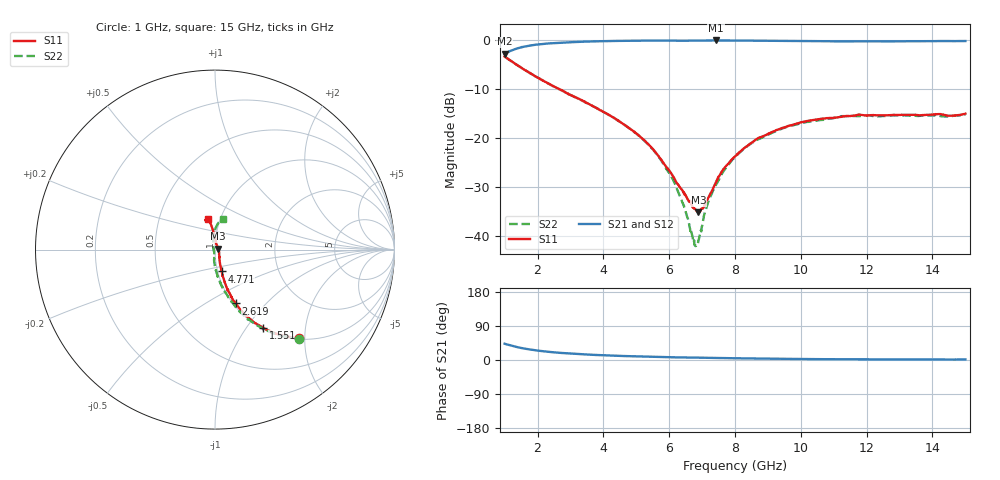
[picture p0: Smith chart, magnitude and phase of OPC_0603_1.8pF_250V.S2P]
! FILE NAME
! DATE 08/20/2012  14:18
! CORRECTED  DATA
# GHz  S  MA  R  50.00
!  FREQ  S11M  S11A  S21M  S21A  S12M  S12A  S22M  S22A
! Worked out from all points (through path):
!   1601 points, 1 GHz to 15 GHz, reference 50 ohm
!   highest |S21| = -0.04 dB at 7.423 GHz (marker M1); lowest = -2.8 dB at 1 GHz (marker M2)
!   group delay of S21, straight-line fit = 5.11 ps
!   lowest |S11| = -35.2 dB at 6.889 GHz (marker M3), VSWR 1.04, Z = 51.7 + j0.571 ohm
!   |S11| at or under -10 dB: 2.662 GHz to end of sweep
!   |S22| runs from -42.1 to -3.3 dB; largest |S21 - S12| = 0.0078
!   S11 on the Smith chart (normalised r, x): 1 GHz: 1.02, -1.88; 1.551 GHz: 1.02, -1.20; 2.619 GHz: 1.03, -0.69; 4.771 GHz: 1.04, -0.26; 15 GHz: 0.87, +0.31
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1  0.681 -46.6  0.7264 43.0  0.726 43.0  0.6811 -46.8
1.55125  0.5116 -58.4  0.8536 30.9  0.8531 30.9  0.5112 -58.9
2.61875  0.3214 -69.0  0.9408 19.3  0.9402 19.3  0.3204 -71.2
3.33625  0.244 -72.2  0.9649 15.2  0.9642 15.2  0.243 -76.6
4.77125  0.1271 -73.0  0.9878 10.1  0.9876 10.1  0.127 -86.3
5.2875  0.09187 -71.3  0.9913 8.8  0.991 8.8  0.09128 -90.4
5.6725  0.06551 -67.6  0.9929 7.9  0.9926 7.9  0.06464 -94.3
6.215  0.03524 -49.3  0.9906 6.9  0.9899 6.9  0.03141 -98.9
6.4775  0.02602 -31.7  0.9896 6.6  0.9888 6.7  0.01868 -103.9
6.775  0.01895 1.4  0.9914 6.3  0.9911 6.4  0.008027 -150.2
6.83625  0.01797 9.5  0.992 6.3  0.9919 6.3  0.007998 -175.5
6.88875  0.0173 18.6  0.9924 6.2  0.992 6.2  0.00896 164.9
7.1425  0.02306 57.7  0.9934 5.8  0.993 5.9  0.01994 116.9
7.4225  0.03526 79.8  0.9951 5.3  0.9935 5.4  0.03319 105.7
7.65  0.04814 84.9  0.9941 5.1  0.9932 5.1  0.04581 102.5
8  0.06485 90.3  0.9933 4.6  0.9925 4.7  0.06374 98.3
8.72625  0.1008 94.7  0.9907 3.9  0.9902 3.9  0.09763 90.8
9.5225  0.1295 98.1  0.9866 3.1  0.9862 3.1  0.1277 86.9
10.33625  0.1519 99.9  0.9819 2.4  0.9811 2.4  0.1484 82.7
11.22875  0.1645 103.1  0.9735 2.1  0.9733 2.1  0.1674 80.3
12.6725  0.171 107.0  0.971 1.8  0.9709 1.8  0.1685 77.2
15  0.1773 103.5  0.9817 1.5  0.9811 1.6  0.1739 75.9
